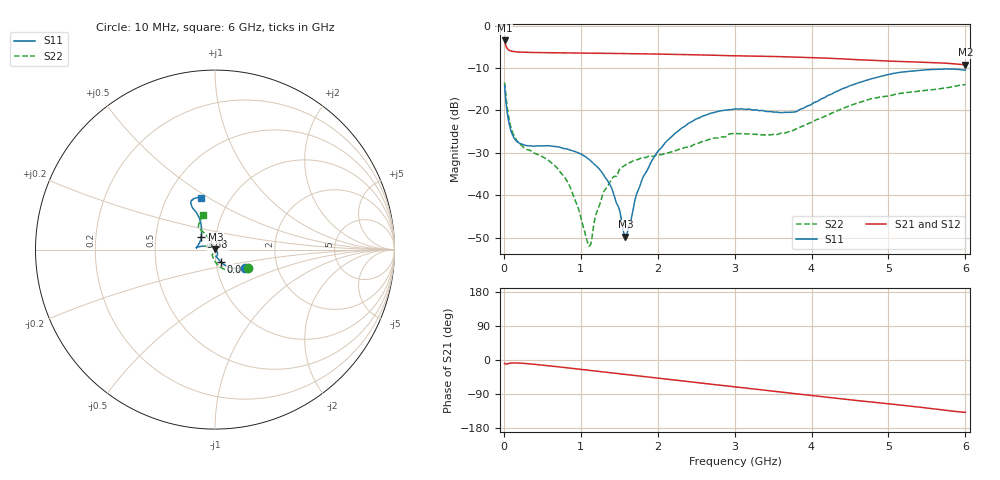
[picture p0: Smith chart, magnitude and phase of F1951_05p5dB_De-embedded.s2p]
! Integrated Device Technology
! Corporate Headquarters
! 6024 Silver Creek Valley Road
! San Jose, CA 95138  USA
! Phone:  1-408-284-8200
! Toll Free:  1-800-223-1366
! Webpage:  http://www.idt.com/
! Timing and RF Division
! 515 Groton Road, Suite 102
! Westford, MA 01886-6024
! Device:  F1951
! Description: 6-bit 0.5 dB Digital Step Attenuator
! Frequency:  100.0 -  4000.00 MHz
! Package:  4x4 mm Thin QFN Plastic Package: 24 pin
! Ports:  2 RF, 6 DC
!  Pin  1  = NC
!  Pin  2  = RF1  =  Port 1
!  Pin  3  = GND
!  Pin  4  = NC
!  Pin  5  = Serial Data Out (SDO)
!  Pin  6  = NC
!  Pin  7  = Reset Bar ( RSTb)
!  Pin  8  = Clock (CLK)
!  Pin  9  = Chip Select Bar (CSb)
!  Pin 10  = NC
!  Pin 11  = Serial Data In (SDI)
!  Pin 12  = NC
!  Pin 13  = NC
!  Pin 14  = VDD
!  Pin 15  = NC
!  Pin 16  = GND
!  Pin 17  = RF2  =  Port 2
!  Pin 18  = NC
!  Pin 19  = GND
!  Pin 20  = GND
!  Pin 21  = GND
!  Pin 22  = GND
!  Pin 23  = GND
!  Pin 24  = GND
! State:  11
! Atten State:  5.5 dB
! Voltage:  +3.30 Volts
! Current:  0.486 mA
! Data:  The device was measured on a F195X evaluation board which has
!  individual transmission lines to the RF pins.  Data was collected
!  de-embedded using a Automatic Fixture Removal [AFR] (Keysight Technologies).
!  The reference plane is the edge of the package pin.
! Misc:  Lot Code  1225BCA
!  Action Tracker AT0399
! Date Measured:  2018-09-13
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# GHz S dB R 50
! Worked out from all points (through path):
!   600 points, 10 MHz to 6 GHz, reference 50 ohm
!   highest |S21| = -3.50 dB at 10 MHz (marker M1); lowest = -9.2 dB at 6 GHz (marker M2)
!   group delay of S21, straight-line fit = 62.8 ps
!   lowest |S11| = -49.8 dB at 1.58 GHz (marker M3), VSWR 1.01, Z = 50.3 + j0.202 ohm
!   |S11| at or under -10 dB: start of sweep to end of sweep
!   |S22| runs from -52.0 to -13.4 dB; largest |S21 - S12| = 0.00064
!   S11 on the Smith chart (normalised r, x): 10 MHz: 1.37, -0.29; 60 MHz: 1.06, -0.15; 3.88 GHz: 0.85, +0.12; 6 GHz: 0.73, +0.46
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0.01  -14.11 -30.9  -3.50 -8.7  -3.50 -8.6  -13.42 -29.3
0.06  -22.34 -64.5  -5.71 -9.2  -5.71 -9.2  -21.23 -79.2
0.12  -26.07 -73.1  -6.10 -7.7  -6.10 -7.7  -25.44 -98.1
0.21  -27.81 -79.3  -6.24 -8.2  -6.24 -8.2  -27.96 -110.7
0.7  -28.58 -76.1  -6.42 -17.8  -6.41 -17.9  -33.74 -113.7
0.85  -29.28 -69.6  -6.45 -21.2  -6.45 -21.2  -37.63 -107.8
1.01  -30.35 -61.9  -6.49 -24.8  -6.49 -24.8  -45.91 -81.8
1.08  -31.18 -59.6  -6.50 -26.3  -6.50 -26.3  -50.66 -40.5
1.12  -31.75 -57.4  -6.51 -27.2  -6.51 -27.2  -51.87 9.4
1.2  -33.07 -53.4  -6.52 -29.0  -6.52 -29.0  -44.41 52.6
1.3  -35.35 -46.3  -6.53 -31.3  -6.53 -31.3  -39.13 65.8
1.41  -38.77 -33.7  -6.56 -33.9  -6.56 -33.9  -35.97 72.4
1.58  -49.82 38.6  -6.60 -37.7  -6.60 -37.7  -32.89 81.5
1.79  -36.68 132.8  -6.65 -42.7  -6.65 -42.7  -31.19 91.9
2.01  -29.50 150.7  -6.71 -47.9  -6.72 -47.8  -30.41 107.7
2.49  -22.11 166.4  -6.89 -59.1  -6.89 -59.1  -27.95 144.9
3.01  -19.65 174.3  -7.10 -71.0  -7.11 -71.0  -25.43 157.8
3.54  -20.38 160.6  -7.29 -83.1  -7.30 -83.1  -25.69 138.0
3.88  -19.57 137.8  -7.47 -90.9  -7.47 -90.9  -23.73 123.8
4.01  -18.43 128.7  -7.54 -94.0  -7.54 -94.0  -22.76 121.2
5.01  -11.51 118.3  -8.38 -115.8  -8.38 -115.8  -16.60 126.6
6  -10.50 105.6  -9.23 -138.1  -9.24 -138.1  -13.89 108.6
